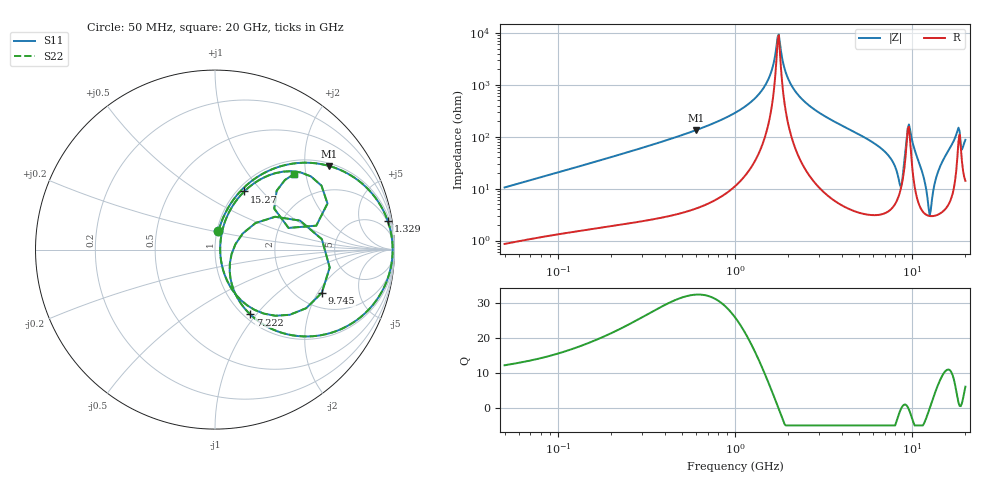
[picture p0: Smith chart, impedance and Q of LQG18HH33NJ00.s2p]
!Murata Part Number: LQG18HH33NJ00
!These Parameters are Measured in Series Mode Connection
!  o--[Z]--o
!Port1  Port2
!  o-------o
!Freq. Start=50[MHz] Stop=20[GHz], 401[Steps]
# Hz S RI R 50
!Freq.(Hz) S11(Real) S11(Imag) S21(Real) S21(Imag) S12(Real) S12(Imag) S22(Real) S22(Imag)
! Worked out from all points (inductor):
!   401 points, 50 MHz to 20 GHz, reference 50 ohm
!   read as one part in series: L = 33.1 nH near 51.52 MHz
!   highest Q = 32.4 at 600.9 MHz (marker M1), where L = 35.4 nH
!   self-resonance near 1.741 GHz
!   S11 on the Smith chart (normalised r, x): 50 MHz: 1.02, +0.21; 1.329 GHz: 2, +12; 7.222 GHz: 1.07, -0.93; 9.745 GHz: 2.65, -2.17; 15.27 GHz: 1.08, +0.80; 20 GHz: 1.28, +1.72
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5e7  0.0192 0.1022  0.9808 -0.1022  0.9808 -0.1022  0.0192 0.1022
1.364002e8  0.0836 0.2503  0.9164 -0.2503  0.9164 -0.2503  0.0836 0.2503
3.721004e8  0.3767 0.4674  0.6233 -0.4674  0.6233 -0.4674  0.3767 0.4674
6.009314e8  0.6372 0.4656  0.3628 -0.4656  0.3628 -0.4656  0.6372 0.4656
1e9  0.8835 0.3022  0.1165 -0.3022  0.1165 -0.3022  0.8835 0.3022
1.329223e9  0.9629 0.1583  0.0371 -0.1583  0.0371 -0.1583  0.9629 0.1583
1.567309e9  0.9851 0.0663  0.0149 -0.0663  0.0149 -0.0663  0.9851 0.0663
1.766834e9  0.9898 -0.00268  0.0102 0.00268  0.0102 0.00268  0.9898 -0.00268
2.05233e9  0.9815 -0.0899  0.0185 0.0899  0.0185 0.0899  0.9815 -0.0899
2.728004e9  0.9193 -0.2523  0.0807 0.2523  0.0807 0.2523  0.9193 -0.2523
4.89267e9  0.5711 -0.4799  0.4289 0.4799  0.4289 0.4799  0.5711 -0.4799
7.222371e9  0.1966 -0.3614  0.8034 0.3614  0.8034 0.3614  0.1966 -0.3614
7.442007e9  0.1675 -0.3305  0.8325 0.3305  0.8325 0.3305  0.1675 -0.3305
8.644534e9  0.0919 -0.0266  0.9081 0.0266  0.9081 0.0266  0.0919 -0.0266
9.178299e9  0.335 0.183  0.665 -0.183  0.665 -0.183  0.335 0.183
9.745021e9  0.5952 -0.2405  0.4048 0.2405  0.4048 0.2405  0.5952 -0.2405
1.019291e10  0.3366 -0.3686  0.6634 0.3686  0.6634 0.3686  0.3366 -0.3686
1.131968e10  0.0799 -0.1976  0.9201 0.1976  0.9201 0.1976  0.0799 -0.1976
1.257102e10  0.0288 -0.00253  0.9712 0.00253  0.9712 0.00253  0.0288 -0.00253
1.527346e10  0.1632 0.3241  0.8368 -0.3241  0.8368 -0.3241  0.1632 0.3241
1.800918e10  0.5934 0.3561  0.4066 -0.3561  0.4066 -0.3561  0.5934 0.3561
2e10  0.4416 0.4213  0.5584 -0.4213  0.5584 -0.4213  0.4416 0.4213
